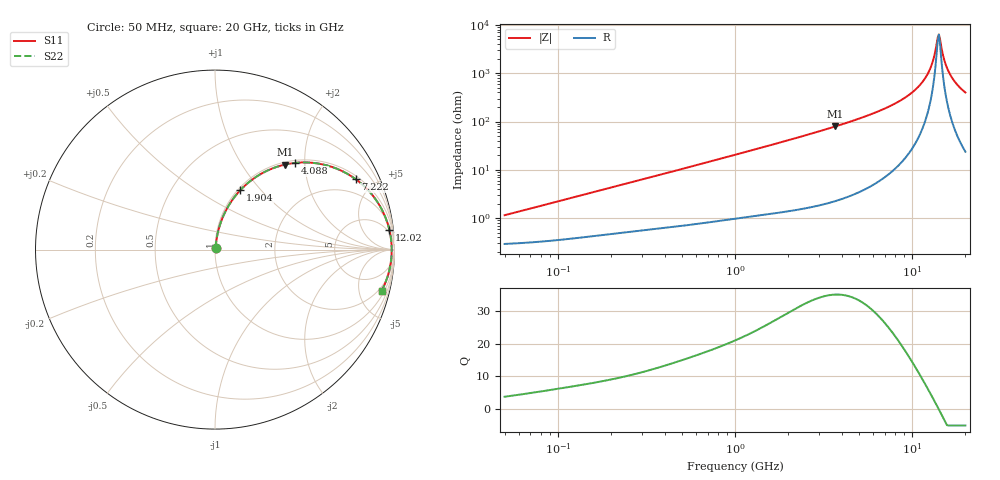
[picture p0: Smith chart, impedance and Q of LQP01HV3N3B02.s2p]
!Murata Part Number: LQP01HV3N3B02
!These Parameters are Measured in Series Mode Connection
!  o--[Z]--o
!Port1  Port2
!  o-------o
!Freq. Start=50[MHz] Stop=20[GHz], 401[Steps]
# Hz S RI R 50
!Freq.(Hz) S11(Real) S11(Imag) S21(Real) S21(Imag) S12(Real) S12(Imag) S22(Real) S22(Imag)
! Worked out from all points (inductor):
!   401 points, 50 MHz to 20 GHz, reference 50 ohm
!   read as one part in series: L = 3.54 nH near 51.52 MHz
!   highest Q = 35.1 at 3.681 GHz (marker M1), where L = 3.42 nH
!   self-resonance near 13.96 GHz
!   S11 on the Smith chart (normalised r, x): 50 MHz: 1.01, +0.02; 1.904 GHz: 1.03, +0.78; 4.088 GHz: 1.05, +1.79; 7.222 GHz: 1.15, +3.90; 12.02 GHz: 3, +17; 20 GHz: 1.48, -7.97
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5e7  0.00305 0.0111  0.997 -0.0111  0.997 -0.0111  0.00305 0.0111
1.364002e8  0.00484 0.0294  0.9952 -0.0294  0.9952 -0.0294  0.00484 0.0294
3.721004e8  0.012 0.0764  0.988 -0.0764  0.988 -0.0764  0.012 0.0764
1e9  0.0488 0.1929  0.9512 -0.1929  0.9512 -0.1929  0.0488 0.1929
1.904239e9  0.141 0.3311  0.859 -0.3311  0.859 -0.3311  0.141 0.3311
2.728004e9  0.251 0.4188  0.749 -0.4188  0.749 -0.4188  0.251 0.4188
3.680849e9  0.3882 0.4733  0.6118 -0.4733  0.6118 -0.4733  0.3882 0.4733
4.087748e9  0.4455 0.4829  0.5545 -0.4829  0.5545 -0.4829  0.4455 0.4829
5.433528e9  0.6159 0.4711  0.3841 -0.4711  0.3841 -0.4711  0.6159 0.4711
7.222371e9  0.7834 0.3928  0.2166 -0.3928  0.2166 -0.3928  0.7834 0.3928
7.442007e9  0.7994 0.3807  0.2006 -0.3807  0.2006 -0.3807  0.7994 0.3807
9.892087e9  0.9236 0.2343  0.0764 -0.2343  0.0764 -0.2343  0.9236 0.2343
1.098561e10  0.9535 0.1692  0.0465 -0.1692  0.0465 -0.1692  0.9535 0.1692
1.201863e10  0.9714 0.1104  0.0286 -0.1104  0.0286 -0.1104  0.9714 0.1104
1.295331e10  0.9806 0.06  0.0194 -0.06  0.0194 -0.06  0.9806 0.06
1.375312e10  0.9841 0.0191  0.0159 -0.0191  0.0159 -0.0191  0.9841 0.0191
1.417136e10  0.9845 -0.00146  0.0155 0.00146  0.0155 0.00146  0.9845 -0.00146
1.460232e10  0.9841 -0.022  0.0159 0.022  0.0159 0.022  0.9841 -0.022
1.550395e10  0.9808 -0.0629  0.0192 0.0629  0.0192 0.0629  0.9808 -0.0629
1.621653e10  0.976 -0.0934  0.024 0.0934  0.024 0.0934  0.976 -0.0934
1.774144e10  0.9607 -0.1531  0.0393 0.1531  0.0393 0.1531  0.9607 -0.1531
2e10  0.9289 -0.2289  0.0711 0.2289  0.0711 0.2289  0.9289 -0.2289
